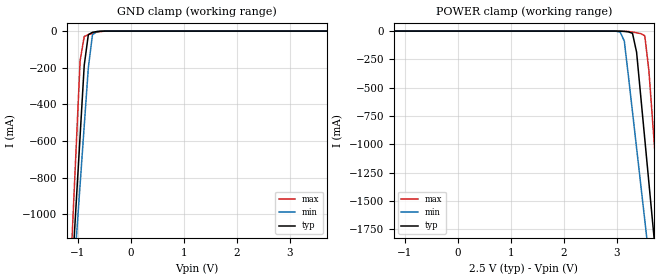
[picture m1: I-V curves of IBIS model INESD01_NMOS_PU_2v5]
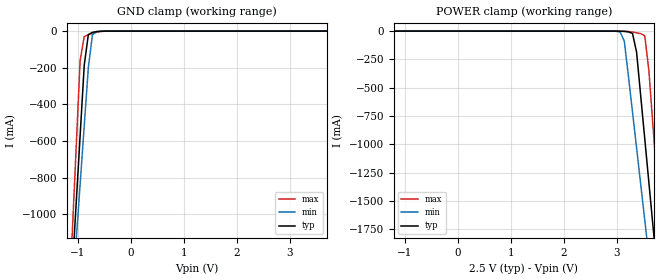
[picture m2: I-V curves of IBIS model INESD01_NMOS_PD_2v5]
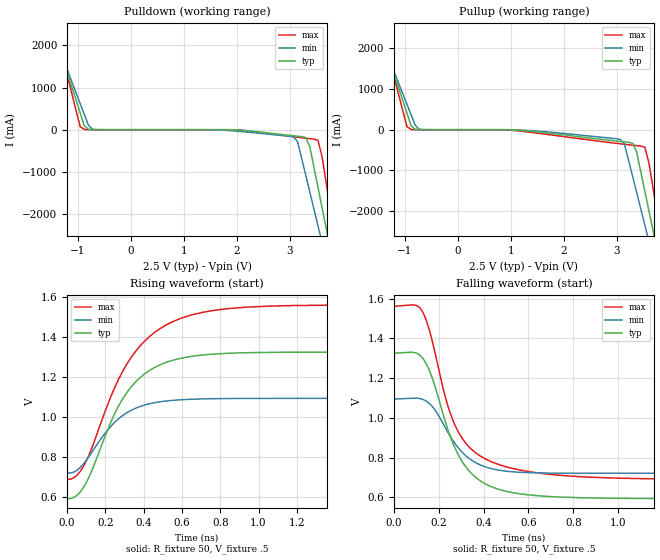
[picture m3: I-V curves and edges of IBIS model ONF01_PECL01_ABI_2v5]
|   This file is an IBIS representation of the   |
|   Integrated Devices Technology, Inc.   |
|   ICS843022I-02   |
|   FEMTOCLOCKS CRYSTAL-TO-3.3V,2.5V LVPECL CLOCK GENERATOR   |
[IBIS Ver]   4.1
[File name]   843022i_02.ibs
[File Rev]   1.0
[Date]   12 Jan 2009 | Last modified
|   Dec 13 2006 | Generated
[Source]   Originated at Integrated Devices Technology, Inc.
[Disclaimer]
IDT hereby grants the user of this IBIS model a non-exclusive,
nontransferable license to use this IBIS model under the following terms.
Before using this IBIS model, the user should read this license.
If the user does not accept these terms,  the IBIS model should be
returned to IDT within 30 days.
   The user is granted this license only to use the IBIS model and
is not granted rights to sell, load, rent, lease or license the IBIS
model in whole or in part, or in modified form to anyone other than
user. User may modify the IBIS model to suit its specific
applications but rights to derivative works and such modifications
shall belong to IDT.
   This IBIS model is provided on an "AS IS" basis and IDT makes
absolutely no warranty with respect to the information contained
herein. IDT DISCLAIMS AND CUSTOMER WAIVES ALL WARRANTIES, EXPRESS
OR IMPLIED, INCLUDING WARRANTIES OF MERCHANTABILITY OR FITNESS FOR
A PARTICULAR PURPOSE. The entire risk as to quality and performance
is with the Customer. ACCORDINGLY, IN NO EVENT SHALL THE COMPANY BE
LIABLE FOR ANY DAMAGES, WHETHER IN CONTRACT OR TORT,INCLUDING ANY
LOST PROFITS OR OTHER INCIDENTAL, CONSEQUENTIAL, EXEMPLARY, OR
PUNITIVE DAMAGES ARISING OUT OF THE USE OR APPLICATION OF THE IBIS
model provided in this package. Further, IDT reserves the right to
make changes without notice to any product herein to improve
reliability, function, or design. IDT does not convey any license
under patent rights or any other intellectual property rights,
including those of third parties.
   IDT is not obligated to provide maintenance or support
for the licensed IBIS model.
[Copyright]   Copyright 2006 by Integrated Device Technology, Inc.
[Component]   ICS843022I-02
[Manufacturer] Integrated Devices Technology, Inc.
[Package]
|LD QFN 16
|lead + wire   typ   min   max
R_pkg   72.4655m   58.886m   86.045m
L_pkg   1.47175nH   1.11650nH   1.77850nH
C_pkg   0.07747pF   0.07444pF   0.08050pF
[Pin] signal_name   model_name   R_pin   L_pin   C_pin
1   PWR_DN   INESD01_NMOS_PU   86.045m   1.77850nH   0.08050pF
2   XTAL_OUT   NC   58.886m   1.11650nH   0.07444pF
3   XTAL_IN   NC   58.886m   1.11650nH   0.07444pF
4   VEE   GND   86.045m   1.77850nH   0.08050pF
5   VEE   GND   86.045m   1.77850nH   0.08050pF
6   NC   NC   58.886m   1.11650nH   0.07444pF
7   FREQ_SEL   INESD01_NMOS_PD   58.886m   1.11650nH   0.07444pF
8   VEE   GND   86.045m   1.77850nH   0.08050pF
9   VCC   POWER   86.045m   1.77850nH   0.08050pF
10  VCCO   POWER   58.886m   1.11650nH   0.07444pF
11  nQ   ONF01_PECL01_ABI   58.886m   1.11650nH   0.07444pF
12  Q   ONF01_PECL01_ABI   86.045m   1.77850nH   0.08050pF
13  NC   NC   86.045m   1.77850nH   0.08050pF
14  NC   NC   58.886m   1.11650nH   0.07444pF
15  NC   NC   58.886m   1.11650nH   0.07444pF
16  VCC   POWER   86.045m   1.77850nH   0.08050pF
[Diff Pin]  inv_pin  vdiff tdelay_typ tdelay_min  tdelay_max
12   11   NA   0  0  0
[Model Selector] INESD01_NMOS_PU
INESD01_NMOS_PU_2v5  Buffer selection for 2v5
INESD01_NMOS_PU_3v3  Buffer selection for 3v3
[Model Selector] INESD01_NMOS_PD
INESD01_NMOS_PD_2v5  Buffer selection for 2v5
INESD01_NMOS_PD_3v3  Buffer selection for 3v3
[Model Selector] ONF01_PECL01_ABI
ONF01_PECL01_ABI_2v5  Buffer selection for 2v5
ONF01_PECL01_ABI_3v3  Buffer selection for 3v3
| Models and submodels in the file (6): INESD01_NMOS_PU_2v5 (Input), INESD01_NMOS_PD_2v5 (Input), ONF01_PECL01_ABI_2v5 (Output_ECL), INESD01_NMOS_PU_3v3 (Input), INESD01_NMOS_PD_3v3 (Input), ONF01_PECL01_ABI_3v3 (Output_ECL)
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[Model] INESD01_NMOS_PU_2v5
Model_type   Input
Polarity   Non-Inverting
Vinl = 0.5V
Vinh = 1.1V
|   typ   min   max
C_comp   2pF   1.5pF   2.5pF
|   typ   min   max
[Voltage range]  2.5V   2.375V   2.625V
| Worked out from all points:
|   GND clamp passes 1 mA (typ) near -0.57 V on its own axis
[GND_clamp]
|Voltage I(typ)   I(min)   I(max)
-2.5V     -8.263A    -7.237A    -9.981A
-1.108V   -1.337A    -1.473A    -1.142A
-1.031V   -953.1mA   -1.154A    -651.2mA
-953.6mV  -569.5mA   -835mA     -160.3mA
-876.3mV  -186.2mA   -516.8mA   -29.47mA
-799mV    -19.59mA   -199.2mA   -19.31mA
-721.6mV  -6.713mA   -20.65mA   -12.35mA
-644.3mV  -2.945mA   -2.694mA   -6.489mA
-489.7mV  -219.7uA   -96.65uA   -544uA
5V        555.4pA    974.3pA    139.3pA
[POWER_clamp]
|Voltage   I(typ)   I(min)   I(max)
-2.5V     555.4pA    852.5pA    162.9pA
3.067V    -971.3uA   -8.981mA   -175.9uA
3.144V    -2.945mA   -87.2mA    -1.018mA
3.299V    -19.59mA   -713mA     -8.571mA
3.376V    -186.2mA   -1.031A    -14.91mA
3.454V    -569.5mA   -1.35A     -22.33mA
3.531V    -953.1mA   -1.669A    -41.51mA
3.608V    -1.337A    -1.989A    -348.5mA
3.686V    -1.721A    -2.309A    -839.4mA
3.763V    -2.106A    -2.628A    -1.33A
3.84V     -2.49A     -2.948A    -1.822A
5V        -8.263A    -7.755A    -9.188A
[Model] INESD01_NMOS_PD_2v5
Model_type   Input
Polarity   Non-Inverting
Vinl = 0.5V
Vinh = 1.1V
|   typ   min   max
C_comp   2pF   1.5pF   2.5pF
|   typ   min   max
[Voltage range]  2.5V   2.375V   2.625V
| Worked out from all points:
|   GND clamp passes 1 mA (typ) near -0.57 V on its own axis
[GND_clamp]
|Voltage I(typ)   I(min)   I(max)
-2.5V     -8.263A    -7.237A    -9.981A
-1.108V   -1.337A    -1.473A    -1.142A
-1.031V   -953.2mA   -1.154A    -651.2mA
-953.6mV  -569.5mA   -835.1mA   -160.4mA
-876.3mV  -186.2mA   -516.9mA   -29.49mA
-799mV    -19.6mA    -199.2mA   -19.32mA
-721.6mV  -6.727mA   -20.67mA   -12.36mA
-644.3mV  -2.958mA   -2.71mA    -6.498mA
-489.7mV  -229.2uA   -108.5uA   -551.4uA
5V        96.94uA    121.2uA    75.12uA
[POWER_clamp]
|Voltage   I(typ)   I(min)   I(max)
-2.5V     96.94uA    118.2uA    76.99uA
3.067V    -982.3uA   -8.998mA   -182.6uA
3.144V    -2.958mA   -87.22mA   -1.026mA
3.299V    -19.6mA    -713mA     -8.581mA
3.376V    -186.2mA   -1.032A    -14.92mA
3.454V    -569.5mA   -1.35A     -22.34mA
3.531V    -953.2mA   -1.669A    -41.52mA
3.608V    -1.337A    -1.989A    -348.5mA
3.686V    -1.721A    -2.309A    -839.4mA
3.763V    -2.106A    -2.628A    -1.33A
3.84V     -2.49A     -2.948A    -1.822A
5V        -8.263A    -7.755A    -9.188A
[Model] ONF01_PECL01_ABI_2v5
Model_type  Output_ECL
Polarity   Non-Inverting
Vmeas = .975
Rref = 50
Cref = 0
Vref = .5
|Variable  typ   min   max
C_comp   2p   1.5p   2.5p
[Voltage Range]   2.5   2.375   2.625
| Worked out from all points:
|   rising waveform, R_fixture 50, V_fixture .5: 20-80 % time 228ps typ, 199ps min, 276ps max; typ from 0.592 V to 1.33 V
|   falling waveform, R_fixture 50, V_fixture .5: 20-80 % time 153ps typ, 140ps min, 156ps max; typ from 1.33 V to 0.592 V
| Open source, no load
|  Voltage   I(typ)   I(min)   I(max)
[Pullup]
-2.5V     6.581A     5.758A     7.966A
-1.572V   2.868A     2.671A     3.219A
-1.418V   2.25A      2.158A     2.429A
-953.6mV  402.1mA    621.9mA    72.14mA
-876.3mV  95.6mA     366.6mA    5.897mA
-721.6mV  951.4uA    9.59mA     751.4uA
3.067V    -287.8mA   -237.7mA   -346mA
3.299V    -330.4mA   -1.134A    -380.1mA
3.531V    -1.506A    -2.34A     -427.9mA
3.686V    -2.47A     -3.144A    -1.427A
3.84V     -3.434A    -3.947A    -2.655A
5V        -10.66A    -9.976A    -11.86A
[Pulldown]
-2.5V     6.581A     5.758A     7.966A
-1.495V   2.559A     2.415A     2.824A
-1.418V   2.25A      2.158A     2.429A
-953.6mV  402.1mA    621.9mA    72.14mA
-876.3mV  95.6mA     366.6mA    5.897mA
-721.6mV  951.4uA    9.59mA     751.4uA
3.067V    -142.9mA   -171.4mA   -166.7mA
3.299V    -185mA     -1.067A    -201.5mA
3.531V    -1.361A    -2.272A    -250mA
3.686V    -2.324A    -3.076A    -1.249A
3.84V     -3.288A    -3.879A    -2.478A
5V        -10.51A    -9.904A    -11.69A
[Ramp]
|   typ   min   max
dV/dt_r   0.586/0.368n   0.299/0.313n   0.698/0.446n
dV/dt_f   0.590/0.258n   0.302/0.226n   0.703/0.290n
R_load =   50.0000
[Rising Waveform]
R_fixture = 50
V_fixture = .5   | VCC_typ - 2V
V_fixture_max = 0.625   | VCC_max - 2V
V_fixture_min = 0.375   | VCC_min - 2V
C_fixture = 0.0p
| Time   typ   min   max
0s        592.5mV    720.8mV    689.3mV
46.2ps    605.5mV    731.1mV    704.8mV
92.4ps    659.4mV    774.5mV    766.4mV
241.5ps   1.003V     967.6mV    1.133V
323.4ps   1.138V     1.029V     1.283V
426.3ps   1.231V     1.066V     1.4V
552.3ps   1.285V     1.084V     1.478V
711.9ps   1.312V     1.092V     1.525V
940.8ps   1.323V     1.094V     1.551V
1.999ns   1.326V     1.094V     1.562V
[Falling Waveform]
R_fixture = 50
V_fixture = .5   | VCC_typ - 2V
V_fixture_max = 0.625   | VCC_max - 2V
V_fixture_min = 0.375   | VCC_min - 2V
C_fixture = 0.0p
| Time   typ   min   max
0s        1.326V     1.094V     1.562V
92.4ps    1.328V     1.099V     1.568V
123.9ps   1.306V     1.095V     1.541V
168ps     1.209V     1.061V     1.4V
231ps     973.8mV    945.4mV    1.097V
277.2ps   835.9mV    862.7mV    951mV
348.6ps   716.5mV    784.8mV    838.7mV
447.3ps   647.2mV    740.6mV    773mV
865.2ps   596.5mV    720.8mV    701.4mV
1.999ns   592.4mV    720.7mV    689.3mV
